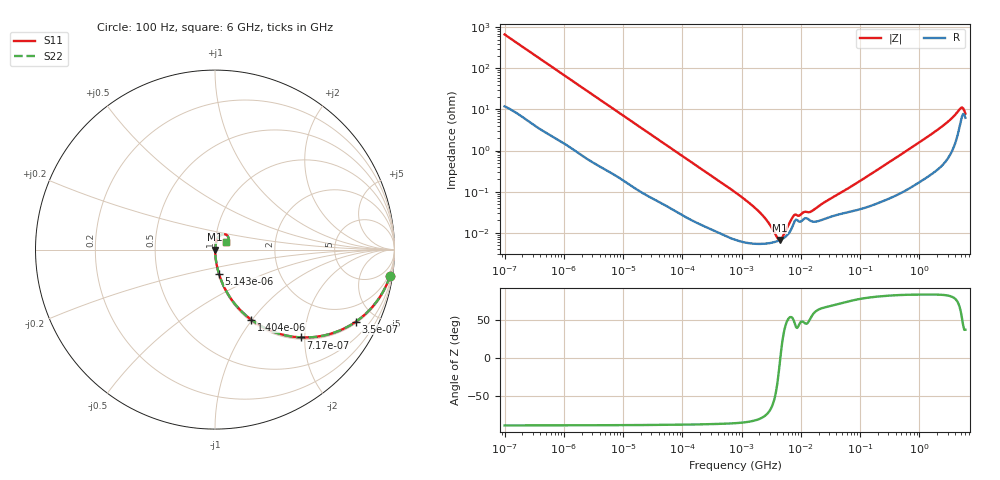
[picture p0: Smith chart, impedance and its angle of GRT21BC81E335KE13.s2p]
!Murata Part Number: GRT21BC81E335KE13
!These Parameters are Measured in Series Mode Connection
!Data Generated on Jun 19, 2026
!  o--ll--o
!Port1  Port2
!  o------o
!Operation Temp=25[degC], DC Bias Voltage=0[V]
!Freq. Start=100[Hz] Stop=6[GHz] 401[Steps]
# Hz S RI R 50
!Freq.(Hz) S11(Real) S11(Imag) S21(Real) S21(Imag) S12(Real) S12(Imag) S22(Real) S22(Imag)
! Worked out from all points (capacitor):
!   401 points, 100 Hz to 6 GHz, reference 50 ohm
!   read as one part in series: C = 2.37 uF near 109 Hz
!   lowest |Z| = 6.66 mohm at 4.441 MHz (marker M1)
!   series resonance near 4.51 MHz, so ESL is about 530 pH
!   S11 on the Smith chart (normalised r, x): 100 Hz: 1, -13; 350 Hz: 1.07, -3.88; 717 Hz: 1.04, -1.91; 1.404 kHz: 1.02, -0.99; 5.143 kHz: 1.01, -0.27; 6 GHz: 1.13, +0.10
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100  0.9757 -0.1455  0.0243 0.1455  0.0243 0.1455  0.9757 -0.1455
205  0.9116 -0.2743  0.0884 0.2743  0.0884 0.2743  0.9116 -0.2743
350  0.786 -0.4006  0.214 0.4006  0.214 0.4006  0.786 -0.4006
717  0.4785 -0.4892  0.5215 0.4892  0.5215 0.4892  0.4785 -0.4892
1404  0.2013 -0.3901  0.7987 0.3901  0.7987 0.3901  0.2013 -0.3901
2008  0.1127 -0.3054  0.8873 0.3054  0.8873 0.3054  0.1127 -0.3054
5143  0.0216 -0.1337  0.9784 0.1337  0.9784 0.1337  0.0216 -0.1337
40335  0.000889 -0.0181  0.9991 0.0181  0.9991 0.0181  0.000889 -0.0181
774597  6.87e-05 -0.000973  0.9999 0.000973  0.9999 0.000973  6.87e-05 -0.000973
1983483  5.37e-05 -0.00032  0.9999 0.00032  0.9999 0.00032  5.37e-05 -0.00032
2594782  5.47e-05 -0.000204  0.9999 0.000204  0.9999 0.000204  5.47e-05 -0.000204
3549919  5.92e-05 -8.55e-05  0.9999 8.55e-05  0.9999 8.55e-05  5.92e-05 -8.55e-05
4440638  6.64e-05 -5.5e-06  0.9999 5.5e-06  0.9999 5.5e-06  6.64e-05 -5.5e-06
5079039  7.37e-05 4.37e-05  0.9999 -4.37e-05  0.9999 -4.37e-05  7.37e-05 4.37e-05
5554849  8.1e-05 7.8e-05  0.9999 -7.8e-05  0.9999 -7.8e-05  8.1e-05 7.8e-05
7599586  0.00017 0.0002  0.9998 -0.0002  0.9998 -0.0002  0.00017 0.0002
1.555665e7  0.000188 0.000284  0.9998 -0.000284  0.9998 -0.000284  0.000188 0.000284
3.124326e8  0.00071 0.0052  0.9993 -0.0052  0.9993 -0.0052  0.00071 0.0052
2.142435e9  0.00477 0.0334  0.9952 -0.0334  0.9952 -0.0334  0.00477 0.0334
4.796499e9  0.0448 0.0859  0.9552 -0.0859  0.9552 -0.0859  0.0448 0.0859
5.245841e9  0.0696 0.0782  0.9304 -0.0782  0.9304 -0.0782  0.0696 0.0782
6e9  0.0611 0.0426  0.9389 -0.0426  0.9389 -0.0426  0.0611 0.0426
